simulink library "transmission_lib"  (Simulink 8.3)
settings: Solver=ode45  StartTime=0.0  StopTime=10.0  RelTol=1e-3
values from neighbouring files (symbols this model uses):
  dual_clutch = class_REVS_dual_clutch    [class_REVS_DCT_transmission.m]
  electric = class_REVS_electric(engine)    [electric_standard_car.m]
  gear = class_REVS_gearbox    [class_REVS_AMT_transmission.m]    (also in class_REVS_AT_transmission.m; class_REVS_CVT_transmission.m)
  torque_converter = class_REVS_torque_converter    [class_REVS_AT_transmission.m]    (also in class_REVS_CVT_transmission.m)
  transmission = class_REVS_AT_transmission    [transmission_6AT.m]    (also in transmission_8DCT.m = class_REVS_DCT_transmission; transmission_CVT.m = class_REVS_CVT_transmission)
undefined symbols (not defined in the file or in its folder): clutch, convert, gear_strategy, InitialSpeed_radps, LoadSource, SpeedSource, Value
libraries: general_lib x129, simulink x57, transmission_lib x50, audit_lib x11
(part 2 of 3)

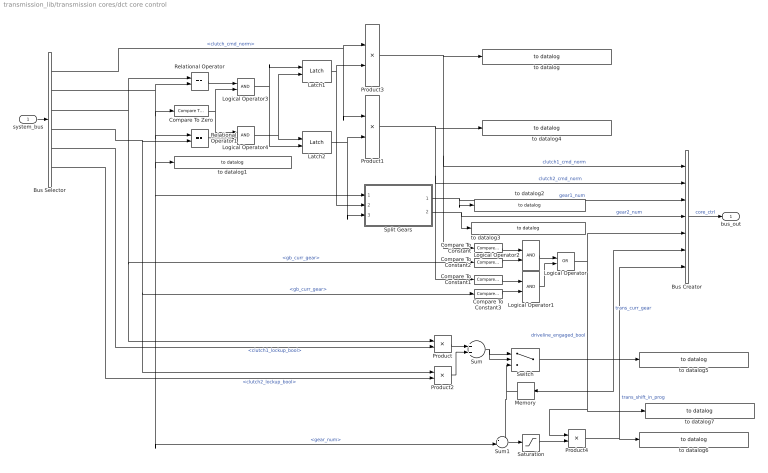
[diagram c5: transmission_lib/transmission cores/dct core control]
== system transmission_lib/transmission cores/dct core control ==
  system_bus : Inport
  Bus Creator : BusCreator  Inputs=7
  Bus Selector : BusSelector  OutputSignals=powertrain.trans.ctrl.clutch_cmd_norm,powertrain.trans.ctrl.gear_num,powertrain.trans.core.gearbox1.gb_curr_gear,powertrain.trans.core.gearbox2.gb_curr_gear,powertrain.trans.core.dual_clutch.clutch1_lockup_bool,powertrain.trans.core.dual_clutch.clutch2_lockup_bool
  Compare To Constant : simulink/Logic and Bit Operations/Compare To Constant  relop=>  const=0.01  OutDataTypeStr=boolean  ZeroCross=off
  Compare To Constant1 : simulink/Logic and Bit Operations/Compare To Constant  relop=>  const=0.01  OutDataTypeStr=boolean  ZeroCross=off
  Compare To Constant2 : simulink/Logic and Bit Operations/Compare To Constant  relop=>  const=0  OutDataTypeStr=boolean  ZeroCross=off
  Compare To Constant3 : simulink/Logic and Bit Operations/Compare To Constant  relop=>  const=0  OutDataTypeStr=boolean  ZeroCross=off
  Compare To Zero : simulink/Logic and Bit Operations/Compare To Zero  relop=~=  OutDataTypeStr=boolean  ZeroCross=off
  Latch1 : general_lib/Latch  tb=On  InitialCondition=0
  Latch2 : general_lib/Latch  tb=On  InitialCondition=0
  Logical Operator : Logic  Operator=OR  AllPortsSameDT=off  OutDataTypeStr=boolean
  Logical Operator{1..4} (4 alike) : Logic  AllPortsSameDT=off  OutDataTypeStr=boolean
  Memory : Memory
  Product{,1..4} (5 alike) : Product
  Relational Operator : RelationalOperator  Operator===  OutDataTypeStr=boolean  ZeroCross=off
  Relational Operator1 : RelationalOperator  Operator===  OutDataTypeStr=boolean  ZeroCross=off
  Saturation : Saturate  UpperLimit=1  LowerLimit=-1  ZeroCross=off
  Split Gears : Subsystem
  Sum : Sum
  Sum1 : Sum  Inputs=-+|
  Switch : Switch  Criteria=u2 > Threshold
  to datalog : general_lib/to datalog  VarName=transmission__clutch1_command_norm  WorkspaceName=datalog__transmission__clutch1_command_norm  VerboseLevel=3  VerboseSignal=REVS.verbose
  to datalog1 : general_lib/to datalog  VarName=transmission__selected_gear_num  WorkspaceName=datalog__transmission__selected_gear_num  VerboseLevel=1  VerboseSignal=REVS.verbose
  to datalog2 : general_lib/to datalog  VarName=transmission__commanded_gear1_num  WorkspaceName=datalog__transmission__commanded_gear1_num  VerboseLevel=1  VerboseSignal=REVS.verbose
  to datalog3 : general_lib/to datalog  VarName=transmission__commanded_gear2_num  WorkspaceName=datalog__transmission__commanded_gear2_num  VerboseLevel=1  VerboseSignal=REVS.verbose
  to datalog4 : general_lib/to datalog  VarName=transmission__clutch2_command_norm  WorkspaceName=datalog__transmission__clutch2_command_norm  VerboseLevel=3  VerboseSignal=REVS.verbose
  to datalog5 : general_lib/to datalog  VarName=transmission__current_gear  WorkspaceName=datalog__transmission__current_gear  VerboseLevel=1  VerboseSignal=REVS.verbose
  to datalog6 : general_lib/to datalog  VarName=transmission.shift_in_progress  WorkspaceName=datalog__transmission__shift_in_progress  VerboseLevel=2  VerboseSignal=REVS.verbose
  to datalog7 : general_lib/to datalog  VarName=transmission__driveline_engaged_bool  WorkspaceName=datalog__transmission__driveline_engaged_bool  VerboseLevel=2  VerboseSignal=REVS.verbose
  bus_out : Outport
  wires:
  Saturation/1 -> Product4/2
  Bus Selector/6 -> Product2/2  "<clutch2_lockup_bool>"
  Bus Selector/5 -> Product/2  "<clutch1_lockup_bool>"
  Sum/1 -> Switch/2, Switch/1
  Product2/1 -> Sum/2
  Product/1 -> Sum/1
  Switch/1 -> Memory/1, to datalog5/1, Bus Creator/6  "trans_curr_gear"
  Product4/1 -> Bus Creator/7, to datalog6/1  "trans_shift_in_prog"
  Latch2/1 -> Product1/2, Split Gears/3(clutch2_status)
  Bus Selector/3 -> Relational Operator/1, Compare To Constant2/1, Product/1  "<gb_curr_gear>"
  Latch1/1 -> Split Gears/2(clutch1_status), Product3/2
  Split Gears/1(gear1_num) -> to datalog2/1, Bus Creator/3  "gear1_num"
  Bus Creator/1 -> bus_out/1  "core_ctrl"
  system_bus/1 -> Bus Selector/1
  Bus Selector/2 -> Relational Operator/2, Compare To Zero/1, Relational Operator1/1, to datalog1/1, Sum1/2, Split Gears/1(target_gear)  "<gear_num>"
  Product1/1 -> to datalog4/1, Compare To Constant1/1, Bus Creator/2  "clutch2_cmd_norm"
  Split Gears/2(gear2_num) -> to datalog3/1, Bus Creator/4  "gear2_num"
  Product3/1 -> to datalog/1, Compare To Constant/1, Bus Creator/1  "clutch1_cmd_norm"
  Logical Operator/1 -> Product4/1, to datalog7/1, Bus Creator/5  "driveline_engaged_bool"
  Bus Selector/4 -> Relational Operator1/2, Compare To Constant3/1, Product2/1  "<gb_curr_gear>"
  Compare To Constant/1 -> Logical Operator2/1
  Compare To Constant1/1 -> Logical Operator1/1
  Logical Operator1/1 -> Logical Operator/2
  Logical Operator2/1 -> Logical Operator/1
  Logical Operator3/1 -> Latch1/1, Latch2/2
  Logical Operator4/1 -> Latch2/1, Latch1/2
  Compare To Constant2/1 -> Logical Operator2/2
  Compare To Constant3/1 -> Logical Operator1/2
  Relational Operator/1 -> Logical Operator3/1
  Relational Operator1/1 -> Logical Operator4/2
  Compare To Zero/1 -> Logical Operator4/1, Logical Operator3/2
  Bus Selector/1 -> Product3/1, Product1/1  "<clutch_cmd_norm>"
  Sum1/1 -> Saturation/1
  Memory/1 -> Sum1/1, Switch/3

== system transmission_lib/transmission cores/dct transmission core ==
  trans_bus : Inport
  trq_in_Nm : Inport  Port=2
  iner_in_kgm2 : Inport  Port=3
  spd_out_radps : Inport  Port=4
  Bus Creator : BusCreator  Inputs=5
  Sum : Sum  Inputs=++|
  Sum1 : Sum  Inputs=++|
  dual clutch module : transmission_lib/transmission components/dual clutch module  ClutchBaseName=dual_clutch  dual_clutch=transmission.dual_clutch  InitialSpeed_radps=0
  gearbox1 : transmission_lib/transmission components/gearbox  GearboxBaseName=gearbox1  gear=transmission.gear1  OutputSignals=gear1_num
  gearbox2 : transmission_lib/transmission components/gearbox  GearboxBaseName=gearbox2  gear=transmission.gear2  OutputSignals=gear2_num
  bus_out : Outport
  trq_out_Nm : Outport  Port=2
  iner_out_kgm2 : Outport  Port=3
  spd_in_radps : Outport  Port=4
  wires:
  dual clutch module/1 -> Bus Creator/1  "dual_clutch"
  gearbox2/1 -> Bus Creator/3  "gearbox2"
  gearbox2/3 -> Sum1/2
  gearbox2/2 -> Sum/2
  Sum/1 -> trq_out_Nm/1
  Sum1/1 -> iner_out_kgm2/1
  dual clutch module/3 -> gearbox1/3
  dual clutch module/2 -> gearbox1/2
  gearbox2/4 -> dual clutch module/5
  dual clutch module/4 -> gearbox2/2
  gearbox1/1 -> Bus Creator/2  "gearbox1"
  gearbox1/2 -> Sum/1
  gearbox1/3 -> Sum1/1
  trans_bus/1 -> gearbox1/1, gearbox2/1, dual clutch module/1
  trq_in_Nm/1 -> dual clutch module/2
  Bus Creator/1 -> bus_out/1  "trans"
  spd_out_radps/1 -> gearbox2/4, Bus Creator/5, gearbox1/4  "trans_spd_out_radps"
  iner_in_kgm2/1 -> dual clutch module/3
  dual clutch module/6 -> spd_in_radps/1, Bus Creator/4  "trans_spd_in_radps"
  gearbox1/4 -> dual clutch module/4
  dual clutch module/5 -> gearbox2/3

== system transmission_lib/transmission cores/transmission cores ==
  note: 1) Only subsystems can be added as variant choices at this level 2) Blocks cannot be connected at this level as connectivity is automatically determined at simulation, based on the active variant
  trans_bus : Inport
  trq_in_Nm : Inport  Port=2
  iner_in_kgm2 : Inport  Port=3
  spd_out_radps : Inport  Port=4
  automatic transmission core : transmission_lib/transmission cores/automatic transmission core  VariantControl=(transmission_type == enum_transmission_type.automatic)
  dct transmission core : transmission_lib/transmission cores/dct transmission core  VariantControl=(transmission_type == enum_transmission_type.DCT)
  bus_out : Outport
  trq_out_Nm : Outport  Port=2
  iner_out_kgm2 : Outport  Port=3
  spd_in_radps : Outport  Port=4

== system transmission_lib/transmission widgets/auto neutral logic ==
  system_bus : Inport
  Bus Selector : BusSelector  OutputSignals=vehicle.veh_spd_mps,driver.accel_anticipate_bool,powertrain.control.ctrl_eng_on,powertrain.engine.eng_spd_radps
  Compare To Constant : simulink/Logic and Bit Operations/Compare To Constant  relop=>=  const=transmission.control.auto_neutral_delay_secs  OutDataTypeStr=boolean
  Compare To Zero4 : simulink/Logic and Bit Operations/Compare To Zero  relop=>  OutDataTypeStr=boolean
  Gain : Gain  Gain=1.5
  Logical Operator1 : Logic  Operator=OR  AllPortsSameDT=off  OutDataTypeStr=boolean
  Logical Operator2 : Logic  Inputs=4  AllPortsSameDT=off  OutDataTypeStr=boolean
  Logical Operator3 : Logic  Operator=NOT  AllPortsSameDT=off  OutDataTypeStr=boolean
  Logical Operator4 : Logic  Inputs=3  AllPortsSameDT=off  OutDataTypeStr=boolean
  Relational Operator : RelationalOperator  Operator=<  OutDataTypeStr=boolean
  auto neutral enable : Constant  Value=transmission.control.auto_neutral_enable
  crank speed : Constant  Value=electric.starter.cranking_speed_radps
  stop time : general_lib/boolean integrator  UpperSaturationLimit=Inf  Normalize=off
  stopped speed : simulink/Logic and Bit Operations/Compare To Constant  relop=<=  const=0.1  OutDataTypeStr=boolean
  to datalog1 : general_lib/to datalog  VarName=transmission__auto_neutral_command_bool  WorkspaceName=datalog__transmission__auto_neutral_command_bool  VerboseLevel=3  VerboseSignal=REVS.verbose
  warmup condition : general_lib/dynamic equation  DynamicExpression=transmission.control.auto_neutral_warmup_condition  DynamicExpressionEval=0
  auto_neutral_bool : Outport
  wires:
  Gain/1 -> Relational Operator/2
  crank speed/1 -> Gain/1
  Bus Selector/4 -> Relational Operator/1  "<eng_spd_radps>"
  Relational Operator/1 -> Logical Operator4/3
  Bus Selector/3 -> Logical Operator4/1  "<ctrl_eng_on>"
  Logical Operator2/1 -> Logical Operator1/1
  Logical Operator4/1 -> Logical Operator1/2
  Bus Selector/2 -> Compare To Zero4/1  "<accel_anticipate_bool>"
  Logical Operator1/1 -> to datalog1/1, auto_neutral_bool/1
  Compare To Constant/1 -> Logical Operator2/2
  Bus Selector/1 -> stopped speed/1  "<veh_spd_mps>"
  Logical Operator3/1 -> Logical Operator2/3
  auto neutral enable/1 -> Logical Operator2/1
  Compare To Zero4/1 -> Logical Operator3/1
  warmup condition/1 -> Logical Operator2/4
  stopped speed/1 -> Logical Operator4/2, stop time/1
  stop time/1 -> Compare To Constant/1
  system_bus/1 -> Bus Selector/1, warmup condition/1

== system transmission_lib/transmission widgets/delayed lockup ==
  engage : Inport
  Compare To Constant1 : simulink/Logic and Bit Operations/Compare To Constant  relop===  const=1  OutDataTypeStr=boolean
  Logical Operator2 : Logic  AllPortsSameDT=off  OutDataTypeStr=boolean
  Memory1 : Memory
  lockup : Outport
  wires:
  Compare To Constant1/1 -> Logical Operator2/2, Memory1/1
  engage/1 -> Compare To Constant1/1
  Memory1/1 -> Logical Operator2/1
  Logical Operator2/1 -> lockup/1

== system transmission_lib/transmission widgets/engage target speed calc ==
  engage : Inport
  final_spd_radps : Inport  Port=2
  current_spd_radps : Inport  Port=3
  Compare To Zero : simulink/Logic and Bit Operations/Compare To Zero  relop=>  OutDataTypeStr=boolean
  Fcn : Fcn  Expr=5*(1-u)^3 + .05
  Product1 : Product  Inputs=**//
  Sum2 : Sum  Inputs=|+-
  engage duration : Constant  Value=Value
  engage_accel_radps2 : Outport
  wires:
  Fcn/1 -> Product1/3
  Sum2/1 -> Product1/2
  engage duration/1 -> Product1/4
  Compare To Zero/1 -> Product1/1
  engage/1 -> Compare To Zero/1, Fcn/1
  final_spd_radps/1 -> Sum2/1
  Product1/1 -> engage_accel_radps2/1
  current_spd_radps/1 -> Sum2/2

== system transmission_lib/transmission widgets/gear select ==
  note: 1) Only subsystems can be added as variant choices at this level 2) Blocks cannot be connected at this level as connectivity is automatically determined at simulation, based on the active variant
  system_bus : Inport
  ALPHAshift : transmission_lib/transmission widgets/gear select variants/ALPHAshift  VariantControl=transmission_gear_select == enum_transmission_gear_select.ALPHAshift  gear_strategy=transmission.gear_strategy
  ALPHAshift_CVT : transmission_lib/transmission widgets/gear select variants/ALPHAshift_CVT  VariantControl=transmission_gear_select == enum_transmission_gear_select.ALPHAshift_CVT
  target_gear : Outport

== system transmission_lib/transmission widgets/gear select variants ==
  ALPHAshift : Subsystem  VariantControl=transmission_control_type == enum_transmission_control_type.autoshift3
  ALPHAshift_CVT : Subsystem  VariantControl=variants_trans_control_externalshift

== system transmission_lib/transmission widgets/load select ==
  system_bus : Inport
  Bus Selector : BusSelector  OutputSignals=driver.driver_acl_norm,engine.eng_load_norm,engine.eng_load_Nm
  Constant1 : Constant  Value=LoadSource
  Constant2 : Constant  Value=0
  Multiport Switch : MultiPortSwitch  DataPortOrder=Specify indices  DataPortIndices={enum_load_source.driver_acl_norm, enum_load_source.engine_load_norm,enum_load_source.driver_acl_pct, enum_load_source.engine_load_pct, enum_load_source.engine_load_Nm}  DataPortForDefault=Additional data port
  acl norm to % : Gain  Gain=100
  load norm to % : Gain  Gain=100
  load : Outport
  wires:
  Constant2/1 -> Multiport Switch/7
  Bus Selector/3 -> Multiport Switch/6  "<eng_load_Nm>"
  Constant1/1 -> Multiport Switch/1
  Multiport Switch/1 -> load/1
  system_bus/1 -> Bus Selector/1
  Bus Selector/1 -> acl norm to %/1, Multiport Switch/2  "<driver_acl_norm>"
  Bus Selector/2 -> Multiport Switch/3, load norm to %/1  "<eng_load_norm>"
  acl norm to %/1 -> Multiport Switch/4
  load norm to %/1 -> Multiport Switch/5

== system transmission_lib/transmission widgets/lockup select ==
  note: 1) Only subsystems can be added as variant choices at this level 2) Blocks cannot be connected at this level as connectivity is automatically determined at simulation, based on the active variant
  gear_number : Inport
  system_bus : Inport  Port=2
  lockup rules uber : transmission_lib/transmission widgets/lockup select variants/lockup rules uber  VariantControl=transmission_lockup_select == enum_transmission_lockup_select.uber_dynamic
  table lockup : transmission_lib/transmission widgets/lockup select variants/table lockup  VariantControl=transmission_lockup_select == enum_transmission_lockup_select.table_lockup
  lockup_cmd : Outport

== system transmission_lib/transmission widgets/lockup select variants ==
  lockup rules uber : Subsystem
  table lockup : Subsystem

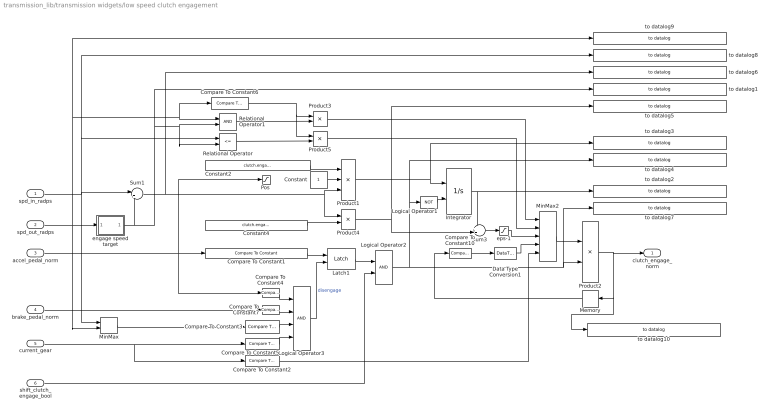
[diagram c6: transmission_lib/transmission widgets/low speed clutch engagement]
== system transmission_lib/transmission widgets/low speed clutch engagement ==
  spd_in_radps : Inport
  spd_out_radps : Inport  Port=2
  accel_pedal_norm : Inport  Port=3
  brake_pedal_norm : Inport  Port=4
  current_gear : Inport  Port=5
  shift_clutch_engage_bool : Inport  Port=6
  Compare To Constant1 : simulink/Logic and Bit Operations/Compare To Constant  relop=>  const=clutch.engage_pedal_norm  OutDataTypeStr=boolean  ZeroCross=off
  Compare To Constant10 : simulink/Logic and Bit Operations/Compare To Constant  relop=>=  const=1  OutDataTypeStr=boolean
  Compare To Constant2 : simulink/Logic and Bit Operations/Compare To Constant  relop=>  const=clutch.engage_modulation_max_gear  OutDataTypeStr=uint8  ZeroCross=off
  Compare To Constant3 : simulink/Logic and Bit Operations/Compare To Constant  relop=<  const=clutch.disengage_speed_radps  OutDataTypeStr=boolean  ZeroCross=off
  Compare To Constant4 : simulink/Logic and Bit Operations/Compare To Constant  relop=<=  const=0  OutDataTypeStr=boolean  ZeroCross=off
  Compare To Constant5 : simulink/Logic and Bit Operations/Compare To Constant  relop=<=  const=clutch.disengage_max_gear  OutDataTypeStr=boolean
  Compare To Constant6 : simulink/Logic and Bit Operations/Compare To Constant  relop=>  const=clutch.engage_speed_radps(1)  OutDataTypeStr=uint8  ZeroCross=off
  Compare To Constant7 : simulink/Logic and Bit Operations/Compare To Constant  relop=>  const=0  OutDataTypeStr=boolean  ZeroCross=off
  Constant : Constant
  Constant2 : Constant  Value=clutch.engage_Ki
  Constant4 : Constant  Value=clutch.engage_Kp
  Data Type Conversion1 : DataTypeConversion  OutDataTypeStr=double
  Integrator : Integrator  ExternalReset=level  LimitOutput=on  UpperSaturationLimit=1  LowerSaturationLimit=0  ZeroCross=off
  Latch1 : general_lib/Latch  tb=Off  InitialCondition=0
  Logical Operator1 : Logic  Operator=NOT  AllPortsSameDT=off  OutDataTypeStr=boolean
  Logical Operator2 : Logic  AllPortsSameDT=off  OutDataTypeStr=boolean
  Logical Operator3 : Logic  Inputs=4  AllPortsSameDT=off  OutDataTypeStr=boolean
  Memory : Memory
  MinMax : MinMax  Function=max  Inputs=2
  MinMax2 : MinMax  Function=max  Inputs=5
  "Pos " : Saturate  UpperLimit=inf  LowerLimit=0  ZeroCross=off
  Product1 : Product  Inputs=3
  Product{2..5} (4 alike) : Product
  Relational Operator : RelationalOperator  Operator=<=  OutDataTypeStr=boolean
  Relational Operator1 : RelationalOperator  OutDataTypeStr=boolean
  Sum1 : Sum  Inputs=|+-
  Sum3 : Sum  Inputs=++|
  engage speed target : Subsystem
  eps-1 : Saturate  UpperLimit=1  LowerLimit=eps  ZeroCross=off
  to datalog1 : general_lib/to datalog  VarName=transmission__clutch_speed_target_radps  WorkspaceName=datalog__transmission__clutch_speed_target_radps  VerboseLevel=2  VerboseSignal=REVS.verbose
  to datalog10 : general_lib/to datalog  VarName=transmission__clutch_engage_norm  WorkspaceName=datalog__transmission__clutch_engage_norm  VerboseLevel=3  VerboseSignal=REVS.verbose
  to datalog2 : general_lib/to datalog  VarName=transmission__clutch_integrator  WorkspaceName=datalog__transmission__clutch_integrator  VerboseLevel=3  VerboseSignal=REVS.verbose
  to datalog3 : general_lib/to datalog  VarName=transmission__clutch_i_term  WorkspaceName=datalog__transmission__clutch_i_term  VerboseLevel=3  VerboseSignal=REVS.verbose
  to datalog4 : general_lib/to datalog  VarName=transmission__clutch_engage_state  WorkspaceName=datalog__transmission__clutch_engage_state  VerboseLevel=3  VerboseSignal=REVS.verbose
  to datalog5 : general_lib/to datalog  VarName=transmission__clutch_p_term  WorkspaceName=datalog__transmission__clutch_p_term  VerboseLevel=3  VerboseSignal=REVS.verbose
  to datalog6 : general_lib/to datalog  VarName=transmission.clutch_speed_error  WorkspaceName=datalog__transmission__clutch_speed_error  VerboseLevel=3  VerboseSignal=REVS.verbose
  to datalog7 : general_lib/to datalog  VarName=transmission__clutch_engage_enable_bool  WorkspaceName=datalog__transmission__clutch_engage_enable_bool  VerboseLevel=3  VerboseSignal=REVS.verbose
  to datalog8 : general_lib/to datalog  VarName=transmission.clutch_speed_in  WorkspaceName=datalog__transmission__clutch_speed_in  VerboseLevel=3  VerboseSignal=REVS.verbose
  to datalog9 : general_lib/to datalog  VarName=transmission.clutch_speed_out  WorkspaceName=datalog__transmission__clutch_speed_out  VerboseLevel=2  VerboseSignal=REVS.verbose
  clutch_engage_norm : Outport
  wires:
  Compare To Constant6/1 -> Product3/1, Product5/1
  Relational Operator1/1 -> Product3/2
  Constant/1 -> Product1/2
  Product3/1 -> MinMax2/1
  Product5/1 -> MinMax2/2
  Relational Operator/1 -> Product5/2
  engage speed target/1(tgt) -> Relational Operator1/2, Relational Operator/2, to datalog1/1, Sum1/2
  spd_out_radps/1 -> engage speed target/1(curr), MinMax/2, Compare To Constant6/1, Relational Operator1/1, to datalog9/1
  accel_pedal_norm/1 -> Compare To Constant4/1, "Pos "/1, Compare To Constant1/1
  MinMax2/1 -> Product2/1
  Compare To Constant3/1 -> Logical Operator3/3
  Constant2/1 -> Product1/1
  Sum1/1 -> Product1/3, Product4/1, to datalog6/1
  "Pos "/1 -> ?
  Logical Operator2/1 -> Logical Operator1/1, to datalog4/1, to datalog7/1, Product2/2
  Product1/1 -> Integrator/1, to datalog3/1
  spd_in_radps/1 -> MinMax/1, Sum1/1, Relational Operator/1, to datalog8/1
  Compare To Constant4/1 -> Logical Operator3/1
  MinMax/1 -> Compare To Constant3/1
  Integrator/1 -> to datalog2/1, Sum3/1
  current_gear/1 -> Compare To Constant5/1, Compare To Constant2/1
  Logical Operator3/1 -> Latch1/2  "disengage"
  Compare To Constant5/1 -> Logical Operator3/4
  Sum3/1 -> eps-1/1
  Product4/1 -> to datalog5/1, Sum3/2
  Compare To Constant2/1 -> MinMax2/5
  brake_pedal_norm/1 -> Compare To Constant7/1
  Compare To Constant7/1 -> Logical Operator3/2
  Constant4/1 -> Product4/2
  Compare To Constant1/1 -> Latch1/1
  Product2/1 -> clutch_engage_norm/1, to datalog10/1, Memory/1
  eps-1/1 -> MinMax2/3
  Compare To Constant10/1 -> Data Type Conversion1/1
  Latch1/1 -> Logical Operator2/1
  Data Type Conversion1/1 -> MinMax2/4
  Memory/1 -> Compare To Constant10/1
  shift_clutch_engage_bool/1 -> Logical Operator2/2
  Logical Operator1/1 -> Integrator/2

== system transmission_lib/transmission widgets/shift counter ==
  target_gear : Inport
  Constant : Constant  Value=transmission.gear.number
  Last Gear : Memory  X0=1
  Memory : Memory  X0=1
  Relational Operator : RelationalOperator  Operator===  OutDataTypeStr=boolean  ZeroCross=off
  Relational Operator1 : RelationalOperator  Operator=>  OutDataTypeStr=boolean  ZeroCross=off
  Relational Operator2 : RelationalOperator  Operator=<  OutDataTypeStr=boolean  ZeroCross=off
  Reshape : Reshape
  Switch : Switch  Criteria=u2 > Threshold
  downshifft result counter : general_lib/result counter  ResultSignalName=num_downshifts  ResultBaseName=''
  result integrator : general_lib/result integrator  ResultSignalName=gear_time_secs  ResultBaseName=''
  uppshift result counter : general_lib/result counter  ResultSignalName=num_upshifts  ResultBaseName=''
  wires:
  Relational Operator1/1 -> uppshift result counter/1
  Constant/1 -> Reshape/1
  Relational Operator/1 -> result integrator/1
  Reshape/1 -> Relational Operator/2
  target_gear/1 -> Relational Operator/1, Switch/1, Switch/2
  Switch/1 -> Last Gear/1, Relational Operator2/1, Relational Operator1/1, Memory/1
  Memory/1 -> Switch/3
  Last Gear/1 -> Relational Operator2/2, Relational Operator1/2
  Relational Operator2/1 -> downshifft result counter/1

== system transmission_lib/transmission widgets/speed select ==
  system_bus : Inport
  Bus Selector : BusSelector  OutputSignals=vehicle.chassis.veh_spd_mps,trans.trans_spd_out_radps,engine.eng_spd_radps,trans.core.trans_spd_in_radps
  Constant : Constant  Value=0
  Constant1 : Constant  Value=SpeedSource
  Multiport Switch : MultiPortSwitch  DataPortOrder=Specify indices  DataPortIndices="{enum_speed_source.vehicle_speed_mph, enum_speed_source.gearbox_output_rpm, enum_speed_source.vehicle_wheel_rpm, enum_speed_source.engine_speed_rpm, enum_speed_source.gearbox_input_rpm, enum_speed_source.gearbox_input_radps, enum_speed_source.gearbox_output_radps, enum_speed_source.engine_speed_radps, enum_speed_source.vehicle_speed_mps,  enum_speed_source.vehicle_speed_kmh}"  DataPortForDefault=Additional data port
  Subsystem : Subsystem
  mps2kmh : Gain  Gain=convert.mps2kmh
  mps2mph : Gain  Gain=convert.mps2mph
  radps2rpm{,1..3} (4 alike) : Gain  Gain=convert.radps2rpm
  spd : Outport
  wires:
  radps2rpm3/1 -> Multiport Switch/6
  Bus Selector/4 -> radps2rpm3/1, Multiport Switch/7  "<trans_spd_in_radps>"
  radps2rpm2/1 -> Multiport Switch/5
  Bus Selector/3 -> radps2rpm2/1, Multiport Switch/9  "<eng_spd_radps>"
  Constant/1 -> Multiport Switch/12
  Bus Selector/1 -> mps2mph/1, mps2kmh/1, Multiport Switch/10, Subsystem/1(veh_spd_mps)  "<veh_spd_mps>"
  Constant1/1 -> Multiport Switch/1
  Multiport Switch/1 -> spd/1
  radps2rpm/1 -> Multiport Switch/3
  Bus Selector/2 -> Multiport Switch/8, radps2rpm/1  "<trans_spd_out_radps>"
  mps2mph/1 -> Multiport Switch/2
  radps2rpm1/1 -> Multiport Switch/4
  system_bus/1 -> Bus Selector/1
  Subsystem/1(wheel_spd_radps) -> radps2rpm1/1
  mps2kmh/1 -> Multiport Switch/11

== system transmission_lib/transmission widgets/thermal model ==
  note: 1) Only subsystems can be added as variant choices at this level 2) Blocks cannot be connected at this level as connectivity is automatically determined at simulation, based on the active variant
  system_bus : Inport
  constant temperature : transmission_lib/transmission widgets/thermal variants/constant temperature  VariantControl=transmission_thermal_type == enum_transmission_thermal_type.constant_temperature
  gradient warmup : transmission_lib/transmission widgets/thermal variants/gradient warmup  VariantControl=transmission_thermal_type == enum_transmission_thermal_type.gradient_temperature
  none : transmission_lib/transmission widgets/thermal variants/none  VariantControl=transmission_thermal_type == enum_transmission_thermal_type.none
  thermal model : transmission_lib/transmission widgets/thermal variants/thermal model  VariantControl=transmission_thermal_type == enum_transmission_thermal_type.thermal_model
  time lookup : transmission_lib/transmission widgets/thermal variants/time lookup  VariantControl=transmission_thermal_type == enum_transmission_thermal_type.time_lookup
  thermal_bus : Outport

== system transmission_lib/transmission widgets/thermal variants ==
  constant temperature : Subsystem
  gradient warmup : Subsystem
  none : Subsystem
  thermal model : Subsystem  VariantControl=transmission_thermal_type == enum_transmission_thermal_type.thermal_model
  time lookup : Subsystem  VariantControl=transmission_thermal_type == enum_transmission_thermal_type.time_lookup

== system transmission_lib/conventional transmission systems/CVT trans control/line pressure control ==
  system_bus : Inport
  Rate Limiter : RateLimiter  RisingSlewLimit=transmission.control.line_press_rate_limit_barps  FallingSlewLimit=-Inf  InitialCondition=3
  dynamic lookup : general_lib/dynamic lookup  LookupStructure=transmission.control.line_pressure_map_bar  InterpMethod=Linear  ExtrapMethod=Clip  DiagnosticForOutOfRangeInput=Warning  IndexSearchMethod=Linear search  BeginIndexSearchUsingPreviousIndexResult=on  SupportTunableTableSize=off  LookupStructureEval=|
      | LookupStructure =
      | 
      |      []
  cmd_line_press_bar : Outport
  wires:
  system_bus/1 -> dynamic lookup/1
  dynamic lookup/1 -> Rate Limiter/1
  Rate Limiter/1 -> cmd_line_press_bar/1

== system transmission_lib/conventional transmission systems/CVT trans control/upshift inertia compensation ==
  system_bus : Inport
  Bus Selector : BusSelector  OutputSignals=powertrain.trans.ctrl.gear_num,powertrain.trans.core.gearbox.gb_curr_gear,powertrain.trans.ctrl.tcc_lockup_cmd_bool,powertrain.trans.trq_conv.tcc_lockup_bool
  Logical Operator : Logic  Operator=OR  AllPortsSameDT=off  OutDataTypeStr=boolean
  Relational Operator : RelationalOperator  Operator=>  OutDataTypeStr=boolean
  Relational Operator1 : RelationalOperator  Operator=>  OutDataTypeStr=boolean
  comp_iner_enable : Outport
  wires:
  Bus Selector/2 -> Relational Operator/2  "<gb_curr_gear>"
  Bus Selector/1 -> Relational Operator/1  "<gear_num>"
  Logical Operator/1 -> comp_iner_enable/1  "eng_comp_iner_enable"
  Bus Selector/3 -> Relational Operator1/1  "<tcc_lockup_cmd_bool>"
  Bus Selector/4 -> Relational Operator1/2  "<tcc_lockup_bool>"
  Relational Operator/1 -> Logical Operator/1
  Relational Operator1/1 -> Logical Operator/2
  system_bus/1 -> Bus Selector/1

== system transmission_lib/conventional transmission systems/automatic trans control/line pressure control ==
  system_bus : Inport
  Rate Limiter : RateLimiter  RisingSlewLimit=transmission.control.line_press_rate_limit_barps  FallingSlewLimit=-Inf  InitialCondition=3
  dynamic lookup : general_lib/dynamic lookup  LookupStructure=transmission.control.line_pressure_map_bar  InterpMethod=Linear  ExtrapMethod=Clip  DiagnosticForOutOfRangeInput=Warning  IndexSearchMethod=Linear search  BeginIndexSearchUsingPreviousIndexResult=on  SupportTunableTableSize=off  LookupStructureEval=|
      | LookupStructure =
      | 
      |      []
  cmd_line_press_bar : Outport
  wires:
  Rate Limiter/1 -> cmd_line_press_bar/1
  dynamic lookup/1 -> Rate Limiter/1
  system_bus/1 -> dynamic lookup/1

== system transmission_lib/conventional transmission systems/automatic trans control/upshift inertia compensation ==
  system_bus : Inport
  Bus Selector : BusSelector  OutputSignals=powertrain.trans.ctrl.gear_num,powertrain.trans.core.gearbox.gb_curr_gear,powertrain.trans.ctrl.tcc_lockup_cmd_bool,powertrain.trans.trq_conv.tcc_lockup_bool
  Logical Operator : Logic  Operator=OR  AllPortsSameDT=off  OutDataTypeStr=boolean
  Relational Operator : RelationalOperator  Operator=>  OutDataTypeStr=boolean
  Relational Operator1 : RelationalOperator  Operator=>  OutDataTypeStr=boolean
  comp_iner_enable : Outport
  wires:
  Bus Selector/2 -> Relational Operator/2  "<gb_curr_gear>"
  Bus Selector/1 -> Relational Operator/1  "<gear_num>"
  Logical Operator/1 -> comp_iner_enable/1  "eng_comp_iner_enable"
  Bus Selector/3 -> Relational Operator1/1  "<tcc_lockup_cmd_bool>"
  Bus Selector/4 -> Relational Operator1/2  "<tcc_lockup_bool>"
  Relational Operator1/1 -> Logical Operator/2
  system_bus/1 -> Bus Selector/1
  Relational Operator/1 -> Logical Operator/1

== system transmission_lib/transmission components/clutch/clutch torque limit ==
  engage : Inport
  "req_transmit_torque_Nm " : Inport  Port=2
  input_speed_radps : Inport  Port=3
  output_speed_radps : Inport  Port=4
  Compare To Constant2 : simulink/Logic and Bit Operations/Compare To Constant  relop=>  const=0  OutDataTypeStr=boolean
  Compare To Zero : simulink/Logic and Bit Operations/Compare To Zero  relop=>=  OutDataTypeStr=boolean  ZeroCross=off
  Compare To Zero1 : simulink/Logic and Bit Operations/Compare To Zero  relop=<=  OutDataTypeStr=boolean  ZeroCross=off
  Constant1 : Constant  Value=-.1
  Constant2 : Constant  Value=.1
  Fcn : Fcn  Expr=u + 1/(100*(1+eps-u))
  Gain : Gain  Gain=-1
  MinMax : MinMax  Function=max  Inputs=2  ZeroCross=off
  MinMax1 : MinMax  Inputs=2  ZeroCross=off
  Product{,1..3} (4 alike) : Product
  Sum : Sum  Inputs=|+-
  Sum1 : Sum  Inputs=|++
  Sum2 : Sum  Inputs=++|
  clutch torque capacity : Constant  Value=transmission.clutch.torque_capacity_Nm
  to datalog1 : general_lib/to datalog  VarName=transmission__clutch_torque_limit_Nm  WorkspaceName=datalog__transmission__clutch_torque_limit_Nm  VerboseLevel=1  VerboseSignal=REVS.verbose
  lim_transmit_torque_Nm : Outport
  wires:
  Compare To Constant2/1 -> Product1/1
  Product1/1 -> lim_transmit_torque_Nm/1
  MinMax/1 -> Product1/2
  Product/1 -> Product3/1, Product2/1, to datalog1/1
  engage/1 -> Compare To Constant2/1, Fcn/1
  Fcn/1 -> Product/1
  clutch torque capacity/1 -> Product/2
  MinMax1/1 -> MinMax/1
  Gain/1 -> Sum1/1
  "req_transmit_torque_Nm "/1 -> MinMax1/1
  input_speed_radps/1 -> Sum/1
  output_speed_radps/1 -> Sum/2
  Constant1/1 -> Sum1/2
  Sum1/1 -> MinMax/2
  Sum/1 -> Compare To Zero1/1, Compare To Zero/1
  Compare To Zero/1 -> Product2/2
  Compare To Zero1/1 -> Product3/2
  Product2/1 -> Sum2/2
  Constant2/1 -> Sum2/1
  Product3/1 -> Gain/1
  Sum2/1 -> MinMax1/2

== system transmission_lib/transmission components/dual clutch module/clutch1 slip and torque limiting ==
  engage : Inport
  input_torque_Nm : Inport  Port=2
  inertia_kgm2 : Inport  Port=3
  input_speed_radps : Inport  Port=4
  output_speed_radps : Inport  Port=5
  Limit Torque : Subsystem
  Product : Product
  Sum2 : Sum  Inputs=+-|
  engage target speed calc : transmission_lib/transmission widgets/engage target speed calc  Value=dual_clutch.engage_duration_secs
  to datalog1 : general_lib/to datalog  VarName=transmission__clutch1_torque_request_Nm  WorkspaceName=datalog__transmission__clutch1_torque_request_Nm  VerboseLevel=3  VerboseSignal=REVS.verbose
  to datalog4 : general_lib/to datalog  VarName=transmission__clutch1_inertia_torque_Nm  WorkspaceName=datalog__transmission__clutch1_inertia_torque_Nm  VerboseLevel=3  VerboseSignal=REVS.verbose
  transmit_torque_Nm : Outport
  torque_limit_Nm : Outport  Port=2
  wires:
  engage/1 -> Limit Torque/1(engage), engage target speed calc/1
  Limit Torque/2(torque_limit_Nm) -> torque_limit_Nm/1
  Sum2/1 -> Limit Torque/2("req_transmit_torque_Nm "), to datalog1/1
  Limit Torque/1(lim_transmit_torque_Nm) -> transmit_torque_Nm/1
  engage target speed calc/1 -> Product/1
  Product/1 -> to datalog4/1, Sum2/2
  inertia_kgm2/1 -> Product/2
  output_speed_radps/1 -> Limit Torque/4(output_speed_radps), engage target speed calc/2
  input_speed_radps/1 -> Limit Torque/3(input_speed_radps), engage target speed calc/3
  input_torque_Nm/1 -> Sum2/1

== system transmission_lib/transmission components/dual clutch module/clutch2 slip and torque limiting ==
  engage : Inport
  input_torque_Nm : Inport  Port=2
  inertia_kgm2 : Inport  Port=3
  input_speed_radps : Inport  Port=4
  output_speed_radps : Inport  Port=5
  Limit Torque : Subsystem
  Product : Product
  Sum2 : Sum  Inputs=+-|
  engage target speed calc : transmission_lib/transmission widgets/engage target speed calc  Value=dual_clutch.engage_duration_secs
  to datalog1 : general_lib/to datalog  VarName=transmission__clutch2_torque_request_Nm  WorkspaceName=datalog__transmission__clutch2_torque_request_Nm  VerboseLevel=3  VerboseSignal=REVS.verbose
  to datalog4 : general_lib/to datalog  VarName=transmission__clutch2_inertia_torque_Nm  WorkspaceName=datalog__transmission__clutch2_inertia_torque_Nm  VerboseLevel=3  VerboseSignal=REVS.verbose
  transmit_torque_Nm : Outport
  torque_limit_Nm : Outport  Port=2
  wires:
  engage/1 -> Limit Torque/1(engage), engage target speed calc/1
  Limit Torque/2(torque_limit_Nm) -> torque_limit_Nm/1
  Sum2/1 -> Limit Torque/2("req_transmit_torque_Nm "), to datalog1/1
  Limit Torque/1(lim_transmit_torque_Nm) -> transmit_torque_Nm/1
  engage target speed calc/1 -> Product/1
  Product/1 -> Sum2/2, to datalog4/1
  inertia_kgm2/1 -> Product/2
  output_speed_radps/1 -> Limit Torque/4(output_speed_radps), engage target speed calc/2
  input_speed_radps/1 -> Limit Torque/3(input_speed_radps), engage target speed calc/3
  input_torque_Nm/1 -> Sum2/1

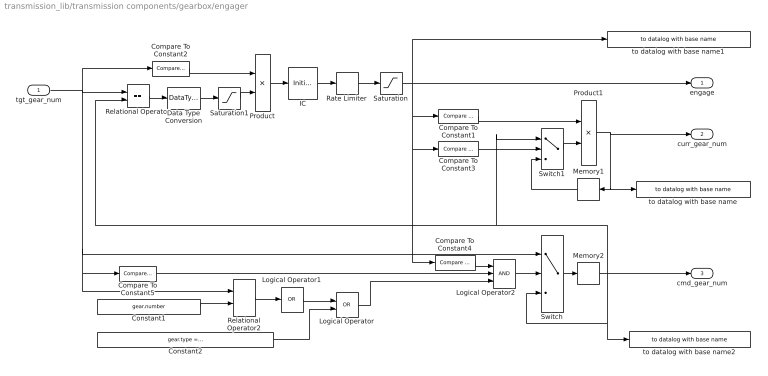
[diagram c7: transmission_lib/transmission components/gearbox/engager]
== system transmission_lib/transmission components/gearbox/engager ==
  tgt_gear_num : Inport
  Compare To Constant1 : simulink/Logic and Bit Operations/Compare To Constant  relop=>  const=0  OutDataTypeStr=boolean  ZeroCross=off
  Compare To Constant2 : simulink/Logic and Bit Operations/Compare To Constant  relop=~=  const=0  OutDataTypeStr=boolean
  Compare To Constant3 : simulink/Logic and Bit Operations/Compare To Constant  relop=>=  const=1  OutDataTypeStr=boolean  ZeroCross=off
  Compare To Constant4 : simulink/Logic and Bit Operations/Compare To Constant  relop=~=  const=1  OutDataTypeStr=boolean  ZeroCross=off
  Compare To Constant5 : simulink/Logic and Bit Operations/Compare To Constant  relop=~=  const=0  OutDataTypeStr=boolean
  Constant1 : Constant  Value=gear.number
  Constant2 : Constant  Value=gear.type == enum_transmission_type.CVT
  Data Type Conversion : DataTypeConversion  OutDataTypeStr=double
  IC : InitialCondition  Value=0
  Logical Operator : Logic  Operator=OR  AllPortsSameDT=off  OutDataTypeStr=boolean
  Logical Operator1 : Logic  Operator=OR  Inputs=1  AllPortsSameDT=off  OutDataTypeStr=boolean
  Logical Operator2 : Logic  Inputs=3  AllPortsSameDT=off  OutDataTypeStr=boolean
  Memory1 : Memory  X0=gear.number(2)
  Memory2 : Memory  X0=gear.number(2)
  Product : Product
  Product1 : Product
  Rate Limiter : RateLimiter  RisingSlewLimit=1/gear.shift_duration_secs  FallingSlewLimit=-inf  InitialCondition=1
  Relational Operator : RelationalOperator  Operator===  OutDataTypeStr=boolean
  Relational Operator2 : RelationalOperator  Operator===  OutDataTypeStr=boolean
  Saturation : Saturate  UpperLimit=1  LowerLimit=0  ZeroCross=off
  Saturation1 : Saturate  UpperLimit=1 - 0.10 * (gear.type == enum_transmission_type.CVT)  LowerLimit=eps + 0.89 * (gear.type == enum_transmission_type.CVT)  ZeroCross=off
  Switch : Switch  Criteria=u2 > Threshold
  Switch1 : Switch  Criteria=u2 > Threshold
  to datalog with base name : general_lib/to datalog with base name  varName=current_gear  baseName=GearboxBaseName  VerboseLevel=1  VerboseSignal=REVS.verbose
  to datalog with base name1 : general_lib/to datalog with base name  varName=gearbox.engage_norm  baseName=GearboxBaseName  VerboseLevel=3  VerboseSignal=REVS.verbose
  to datalog with base name2 : general_lib/to datalog with base name  varName=command_gear  baseName=GearboxBaseName  VerboseLevel=1  VerboseSignal=REVS.verbose
  engage : Outport
  curr_gear_num : Outport  Port=2
  cmd_gear_num : Outport  Port=3
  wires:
  Logical Operator2/1 -> Switch/2
  Logical Operator/1 -> Logical Operator2/3
  Compare To Constant5/1 -> Logical Operator2/2
  Relational Operator2/1 -> Logical Operator1/1
  Constant1/1 -> Relational Operator2/2
  Compare To Constant3/1 -> Switch1/2
  Product1/1 -> curr_gear_num/1, to datalog with base name/1, Memory1/1
  Compare To Constant4/1 -> Logical Operator2/1
  tgt_gear_num/1 -> Compare To Constant2/1, Switch/1, Compare To Constant5/1, Relational Operator2/1, Relational Operator/1
  Saturation1/1 -> Product/2
  Saturation/1 -> engage/1, Compare To Constant1/1, Compare To Constant4/1, Compare To Constant3/1, to datalog with base name1/1
  Switch/1 -> Memory2/1
  Relational Operator/1 -> Data Type Conversion/1
  Product/1 -> IC/1
  IC/1 -> Rate Limiter/1
  Memory2/1 -> Switch1/1, Relational Operator/2, to datalog with base name2/1, Switch/3, cmd_gear_num/1
  Compare To Constant2/1 -> Product/1
  Data Type Conversion/1 -> Saturation1/1
  Rate Limiter/1 -> Saturation/1
  Memory1/1 -> Switch1/3
  Switch1/1 -> Product1/2
  Compare To Constant1/1 -> Product1/1
  Constant2/1 -> Logical Operator/2
  Logical Operator1/1 -> Logical Operator/1

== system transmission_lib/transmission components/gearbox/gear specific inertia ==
  engage : Inport
  cmd_gear_num : Inport  Port=2
  iner_spd_out_radps : Inport  Port=3
  1-D Lookup Table : Lookup_n-D  NumberOfTableDimensions=1  BreakpointsForDimension1=gear.number  Table=gear.inertia_kgm2  InternalRulePriority=Speed  RndMeth=Simplest
  Derivative : Derivative
  Detect Decrease : simulink/Logic and Bit Operations/Detect Decrease  vinit=0.0  InputProcessing=Inherited  OutDataTypeStr=boolean
  Gain : Gain  Gain=.5/1000
  Gain1 : Gain  Gain=0.5
  Inertia Mech E&P Nm radps : audit_lib/Mech E&P Nm radps0  base_name=gearbox2__inertia_spinup_loss  VerboseSignal=REVS.verbose
  Memory : Memory
  Memory1 : Memory
  Product : Product  Inputs=3
  Product1 : Product
  Product4 : Product
  Product5 : Product
  Saturation : Saturate  UpperLimit=inf  LowerLimit=0
  Sum : Sum  Inputs=|++
  inertia KE loss : audit_lib/Misc Audit Signal  AuditBase=Mechanical  VarName=inertia_KE_loss_kJ  BaseName=GearboxBaseName  WorkspaceName=audit__mech__gearbox2__inertia_KE_loss_kJ  VerboseSignal=REVS.verbose
  iner_trq_out_Nm : Outport
  iner_out_kgm2 : Outport  Port=2
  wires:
  Product1/1 -> Sum/1
  1-D Lookup Table/1 -> Product4/2
  Saturation/1 -> Product5/1
  Derivative/1 -> Saturation/1
  engage/1 -> Detect Decrease/1, Product4/1
  Gain/1 -> Memory/1
  Product/1 -> Gain/1
  Detect Decrease/1 -> Product1/2
  Memory/1 -> Product1/1
  iner_spd_out_radps/1 -> Product/3, Product/2, Inertia Mech E&P Nm radps/2, Product5/2
  Product4/1 -> Derivative/1, Product/1, iner_out_kgm2/1
  Product5/1 -> iner_trq_out_Nm/1, Gain1/1
  Gain1/1 -> Inertia Mech E&P Nm radps/1
  Sum/1 -> Memory1/1, inertia KE loss/1
  Memory1/1 -> Sum/2
  cmd_gear_num/1 -> 1-D Lookup Table/1

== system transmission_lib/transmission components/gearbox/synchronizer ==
  engage : Inport
  sync_trq_in_Nm : Inport  Port=2
  sync_iner_in_kgm2 : Inport  Port=3
  sync_spd_out_radps : Inport  Port=4
  " clutch input speed integrator  (integrate when slipping)" : Integrator  ExternalReset=falling  InitialConditionSource=external  LimitOutput=on  UpperSaturationLimit=Inf  LowerSaturationLimit=0
  Clutch Speed Disengaged : Switch  Threshold=1
  IC1 : InitialCondition  Value=0
  Product : Product
  Product2 : Product  Inputs=*/
  Product3 : Product
  Subsystem : Subsystem
  Sum1 : Sum  Inputs=+-|
  Sum2 : Sum  Inputs=+-|
  Torque SW : Switch  Threshold=1
  engage target speed calc : transmission_lib/transmission widgets/engage target speed calc  Value=gear.shift_duration_secs
  synchro limit torque : Subsystem
  to datalog with base name : general_lib/to datalog with base name  varName=gear_synchronizer_lockup  baseName=GearboxBaseName  VerboseLevel=2  VerboseSignal=REVS.verbose
  to datalog with base name1 : general_lib/to datalog with base name  varName=synchronizer_transmit_torque_Nm  baseName=GearboxBaseName  VerboseLevel=2  VerboseSignal=REVS.verbose
  to datalog with base name2 : general_lib/to datalog with base name  varName=synchronizer_engage_torque_Nm  baseName=GearboxBaseName  VerboseLevel=2  VerboseSignal=REVS.verbose
  sync_trq_out_Nm : Outport
  sync_iner_out_kgm2 : Outport  Port=2
  sync_spd_in_radps : Outport  Port=3
  sync_lockup : Outport  Port=4
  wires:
  Subsystem/1(lockup) -> Torque SW/2, Product3/2, Clutch Speed Disengaged/2, sync_lockup/1, " clutch input speed integrator  (integrate when slipping)"/2, to datalog with base name/1
  Clutch Speed Disengaged/1 -> engage target speed calc/3, Subsystem/3(spd_in), synchro limit torque/3(input_speed_radps), sync_spd_in_radps/1
  sync_spd_out_radps/1 -> Clutch Speed Disengaged/1, engage target speed calc/2, IC1/1, synchro limit torque/4(output_speed_radps), Subsystem/2(spd_out)
  engage/1 -> synchro limit torque/1(engage), Subsystem/1(engage), engage target speed calc/1
  Sum1/1 -> Product2/1
  Sum2/1 -> synchro limit torque/2("req_transmit_torque_Nm ")
  engage target speed calc/1 -> Product/1
  sync_iner_in_kgm2/1 -> Product2/2, Product/2, Product3/1
  IC1/1 -> " clutch input speed integrator  (integrate when slipping)"/3
  sync_trq_in_Nm/1 -> Torque SW/1, Sum1/1, Sum2/1
  " clutch input speed integrator  (integrate when slipping)"/1 -> Clutch Speed Disengaged/3
  Product/1 -> to datalog with base name2/1, Sum2/2
  Torque SW/1 -> sync_trq_out_Nm/1
  Product3/1 -> sync_iner_out_kgm2/1
  synchro limit torque/1(lim_transmit_torque_Nm) -> Torque SW/3, to datalog with base name1/1, Sum1/2
  Product2/1 -> " clutch input speed integrator  (integrate when slipping)"/1

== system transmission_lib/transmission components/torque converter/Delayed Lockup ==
  Engage : Inport
  Compare To Constant : simulink/Logic and Bit Operations/Compare To Constant  relop=>  const=0.9  OutDataTypeStr=boolean
  Compare To Constant1 : simulink/Logic and Bit Operations/Compare To Constant  relop=>=  const=1  OutDataTypeStr=boolean
  Logical Operator2 : Logic  AllPortsSameDT=off  OutDataTypeStr=boolean
  Memory1 : Memory
  Lockup : Outport
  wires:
  Compare To Constant1/1 -> Memory1/1
  Compare To Constant/1 -> Logical Operator2/2
  Engage/1 -> Compare To Constant1/1, Compare To Constant/1
  Memory1/1 -> Logical Operator2/1
  Logical Operator2/1 -> Lockup/1

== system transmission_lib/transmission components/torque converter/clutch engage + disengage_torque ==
  engage : Inport
  trq_in_Nm : Inport  Port=2
  final_spd_radps : Inport  Port=3
  current_spd_radps : Inport  Port=4
  iner_in_kgm2 : Inport  Port=5
  Detect Increase : simulink/Logic and Bit Operations/Detect Increase  vinit=0.0  InputProcessing=Inherited  OutDataTypeStr=boolean
  Product1 : Product
  Sum : Sum  Inputs=+-|
  engage target speed calc : transmission_lib/transmission widgets/engage target speed calc  Value=transmission.torque_converter.lockup_duration_secs
  engage trq : Product  Inputs=3
  tcc_torque_Nm : Outport
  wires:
  engage target speed calc/1 -> engage trq/2
  Detect Increase/1 -> engage trq/1
  engage trq/1 -> Sum/2
  Sum/1 -> tcc_torque_Nm/1
  iner_in_kgm2/1 -> engage trq/3
  Product1/1 -> Sum/1
  trq_in_Nm/1 -> Product1/2
  engage/1 -> Product1/1, Detect Increase/1, engage target speed calc/1
  final_spd_radps/1 -> engage target speed calc/2
  current_spd_radps/1 -> engage target speed calc/3

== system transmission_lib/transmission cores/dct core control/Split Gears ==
  note: This formula keeps the gearboxes engaged in the lower gear enabling "immediate" downshifts
  target_gear : Inport
  clutch1_status : Inport  Port=2
  clutch2_status : Inport  Port=3
  Bias : Bias  Bias=-1
  Compare To Zero1 : simulink/Logic and Bit Operations/Compare To Zero  relop=>  OutDataTypeStr=boolean  ZeroCross=off
  Gain : Gain  Gain=0.5
  Gain1 : Gain  Gain=2
  Gain2 : Gain  Gain=2
  Memory : Memory
  Memory1 : Memory
  Product : Product
  Product1 : Product
  Rounding Function : Rounding
  Rounding Function1 : Rounding  Operator=ceil
  Saturation : Saturate  UpperLimit=Inf  LowerLimit=1  ZeroCross=off
  Saturation1 : Saturate  UpperLimit=Inf  LowerLimit=2  ZeroCross=off
  Switch1 : Switch  Criteria=u2 > Threshold
  "Switch2 " : Switch  Criteria=u2 > Threshold
  gear1_num : Outport
  gear2_num : Outport  Port=2
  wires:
  Gain/1 -> Rounding Function1/1, Rounding Function/1
  target_gear/1 -> Compare To Zero1/1, Gain/1
  Rounding Function1/1 -> Gain1/1
  Rounding Function/1 -> Gain2/1
  Gain1/1 -> Bias/1
  Gain2/1 -> Saturation1/1
  Bias/1 -> Saturation/1
  Compare To Zero1/1 -> Product/1, Product1/1
  Saturation/1 -> Switch1/3
  Saturation1/1 -> "Switch2 "/3
  Switch1/1 -> Product/2, Memory/1
  Memory/1 -> Switch1/1
  "Switch2 "/1 -> Product1/2, Memory1/1
  Memory1/1 -> "Switch2 "/1
  clutch1_status/1 -> Switch1/2
  clutch2_status/1 -> "Switch2 "/2
  Product/1 -> gear1_num/1
  Product1/1 -> gear2_num/1
